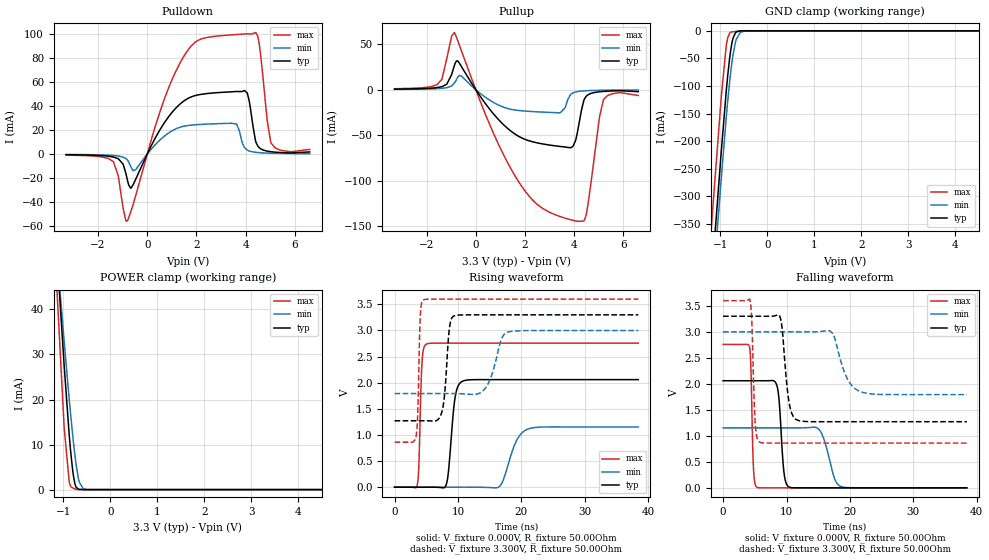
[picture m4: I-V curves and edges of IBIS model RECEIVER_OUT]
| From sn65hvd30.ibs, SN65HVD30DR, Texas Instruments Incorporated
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[Model]   RECEIVER_OUT
Model_type   Output
| Signals   R
Vmeas = 1.3V   |Reference voltage for timing measurements
Cref = 15pF   |Timing specification test load capacitance value
| variable   typ   min   max
C_comp   10.14pF   10.55pF   9.63pF
|   typ   min   max
[Temperature Range]   25.0   -40   85
[Voltage range]   3.3V   3.0V   3.6V
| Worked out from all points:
|   slope of the pulldown table from 0 to 0.495 V, typ, clamps not added: 25.4 ohm
|   slope of the pullup table from 0 to 0.495 V, typ, clamps not added: 26.1 ohm
|   GND clamp passes 1 mA (typ) near -0.61 V on its own axis
|   POWER clamp passes 1 mA (typ) near -0.74 V on its own axis
|   falling waveform, V_fixture 0.000V, R_fixture 50.00Ohm: 20-80 % time 650ps typ, 1.5ns min, 321ps max; typ from 2.06 V to 0.001 V
|   rising waveform, V_fixture 0.000V, R_fixture 50.00Ohm: 20-80 % time 876ps typ, 1.97ns min, 385ps max; typ from 0.001 V to 2.06 V
|   rising waveform, V_fixture 3.300V, R_fixture 50.00Ohm: 20-80 % time 728ps typ, 1.67ns min, 331ps max; typ from 1.27 V to 3.3 V
|   falling waveform, V_fixture 3.300V, R_fixture 50.00Ohm: 20-80 % time 919ps typ, 2.02ns min, 416ps max; typ from 3.3 V to 1.27 V
[Pulldown]
|   Voltage   I(typ)   I(min)   I(max)
-3.3V     -537.3uA   -326.2uA   -829.7uA
-1.376V   -2.454mA   -1.192mA   -6.336mA
-841.8mV  -18.49mA   -4.175mA   -56.13mA
-660.3mV  -28.4mA    -10.81mA   -47.55mA
570.2mV   22.09mA    12.78mA    38.61mA
1.56V     45.3mA     23.56mA    83.98mA
3.631V    52.25mA    25.03mA    99.81mA
3.951V    53.05mA    5.398mA    100.3mA
4.39V     11.83mA    1.507mA    101.4mA
4.544V    5.463mA    1.191mA    92.77mA
5.033V    1.944mA    712.1uA    9.102mA
6.6V      1.793mA    308.2uA    3.898mA
[GND Clamp]
|   Voltage   I(typ)   I(min)   I(max)
-3.3V     -2.763A    -2.767A    -2.713A
-1.376V   -662.8mA   -704.6mA   -567.7mA
-1.178V   -440mA     -485.4mA   -341.4mA
-979.8mV  -219.2mA   -267.9mA   -120mA
-871.9mV  -107.4mA   -155mA     -25.45mA
-841.8mV  -80.52mA   -126.7mA   -12.58mA
-781.8mV  -36.68mA   -77.09mA   -2.596mA
-730.8mV  -13.71mA   -44.15mA   -1.695mA
-660.3mV  -2.029mA   -15.28mA   -877.8uA
-573.4mV  -136.7uA   -2.874mA   -250.4uA
-483.5mV  -8.967uA   -262uA     -45.26uA
6.6V      0A         0A         0A
[Pullup]
|   Voltage   I(typ)   I(min)   I(max)
-3.3V     630.2uA    370.1uA    1.027mA
-1.574V   2.328mA    1.154mA    5.52mA
-871.9mV  26.5mA     7.235mA    62.72mA
-573.2mV  24.94mA    14.77mA    41.96mA
660.7mV   -24.65mA   -13.06mA   -44.23mA
1.758V    -51.44mA   -22.84mA   -101.7mA
3.433V    -62.35mA   -25.31mA   -139.3mA
3.844V    -63.68mA   -5.496mA   -142.7mA
4.134V    -45.79mA   -2.021mA   -144.5mA
4.485V    -7.27mA    -1.116mA   -137.4mA
5.19V     -1.889mA   -580.8uA   -10.72mA
6.6V      -2.127mA   -294.5uA   -6.348mA
[POWER Clamp]
|   Voltage   I(typ)   I(min)   I(max)
-3.3V     431.2mA    345mA      537.7mA
-1.178V   59.35mA    57.84mA    53.2mA
-979.8mV  27.49mA    32.83mA    13.72mA
-871.9mV  11.98mA    19.95mA    1.636mA
-841.8mV  8.418mA    16.6mA     674.6uA
-801.3mV  4.467mA    12.36mA    380.4uA
-752.2mV  1.323mA    7.676mA    163.7uA
-730.8mV  619.1uA    5.883mA    79.78uA
-660.3mV  62.2uA     1.696mA    9.967uA
-573.4mV  2.414uA    158.3uA    354.8nA
-483.5mV  0A         1.987uA    0A
6.6V      0A         0A         0A
[Ramp]
R_load = 50.00Ohm
|   typ   min   max
dV/dt_r   1.216V/728.194ps 723.889mV/1.673ns   1.643V/331.193ps
dV/dt_f   1.235V/649.696ps 691.696mV/1.502ns   1.654V/320.625ps
[Falling Waveform]
V_fixture = 0.000V
V_fixture_min = 0.000V
V_fixture_max = 0.000V
R_fixture = 50.00Ohm
|   Time   V(typ)   V(min)   V(max)
0s        2.059V     1.154V     2.758V
4.187ns   2.059V     1.154V     2.698V
4.814ns   2.059V     1.154V     325.1mV
5.363ns   2.059V     1.154V     9.805mV
8.47ns    1.973V     1.154V     489.2uV
9.565ns   331.4mV    1.154V     492.2uV
10.39ns   17.33mV    1.154V     493.2uV
15.04ns   954.6uV    1.133V     493.5uV
18.57ns   959.7uV    27.47mV    493.4uV
38.43ns   960.9uV    985.2uV    493.4uV
[Rising Waveform]
V_fixture = 0.000V
V_fixture_min = 0.000V
V_fixture_max = 0.000V
R_fixture = 50.00Ohm
|   Time   V(typ)   V(min)   V(max)
0s        960.9uV    985.2uV    493.4uV
3.543ns   960.3uV    985.1uV    21.47mV
4.32ns    957.9uV    985.1uV    2.366V
5.011ns   1.002mV    985.1uV    2.738V
8.104ns   34.13mV    982.6uV    2.758V
9.565ns   1.732V     1.012mV    2.758V
10.58ns   2.02V      1.127mV    2.758V
16.63ns   2.059V     25.52mV    2.758V
21.37ns   2.059V     1.126V     2.758V
38.43ns   2.059V     1.154V     2.758V
[Rising Waveform]
V_fixture = 3.300V
V_fixture_min = 3.000V
V_fixture_max = 3.600V
R_fixture = 50.00Ohm
|   Time   V(typ)   V(min)   V(max)
0s        1.272V     1.792V     861.5mV
3.423ns   1.272V     1.792V     988mV
4.048ns   1.272V     1.792V     3.25V
4.517ns   1.272V     1.792V     3.582V
7.495ns   1.456V     1.792V     3.6V
8.591ns   2.979V     1.793V     3.6V
9.322ns   3.275V     1.793V     3.6V
14.09ns   3.299V     1.861V     3.6V
17.92ns   3.299V     2.971V     3.6V
38.43ns   3.299V     2.999V     3.6V
[Falling Waveform]
V_fixture = 3.300V
V_fixture_min = 3.000V
V_fixture_max = 3.600V
R_fixture = 50.00Ohm
|   Time   V(typ)   V(min)   V(max)
0s        3.299V     2.999V     3.6V
4.247ns   3.299V     2.999V     3.611V
5.087ns   3.299V     2.999V     1.212V
5.769ns   3.299V     2.999V     879.3mV
8.957ns   3.294V     2.999V     861.5mV
10.39ns   1.648V     2.999V     861.5mV
11.61ns   1.309V     2.999V     861.5mV
17.05ns   1.272V     2.999V     861.5mV
22.12ns   1.272V     1.831V     861.5mV
38.43ns   1.272V     1.792V     861.5mV
